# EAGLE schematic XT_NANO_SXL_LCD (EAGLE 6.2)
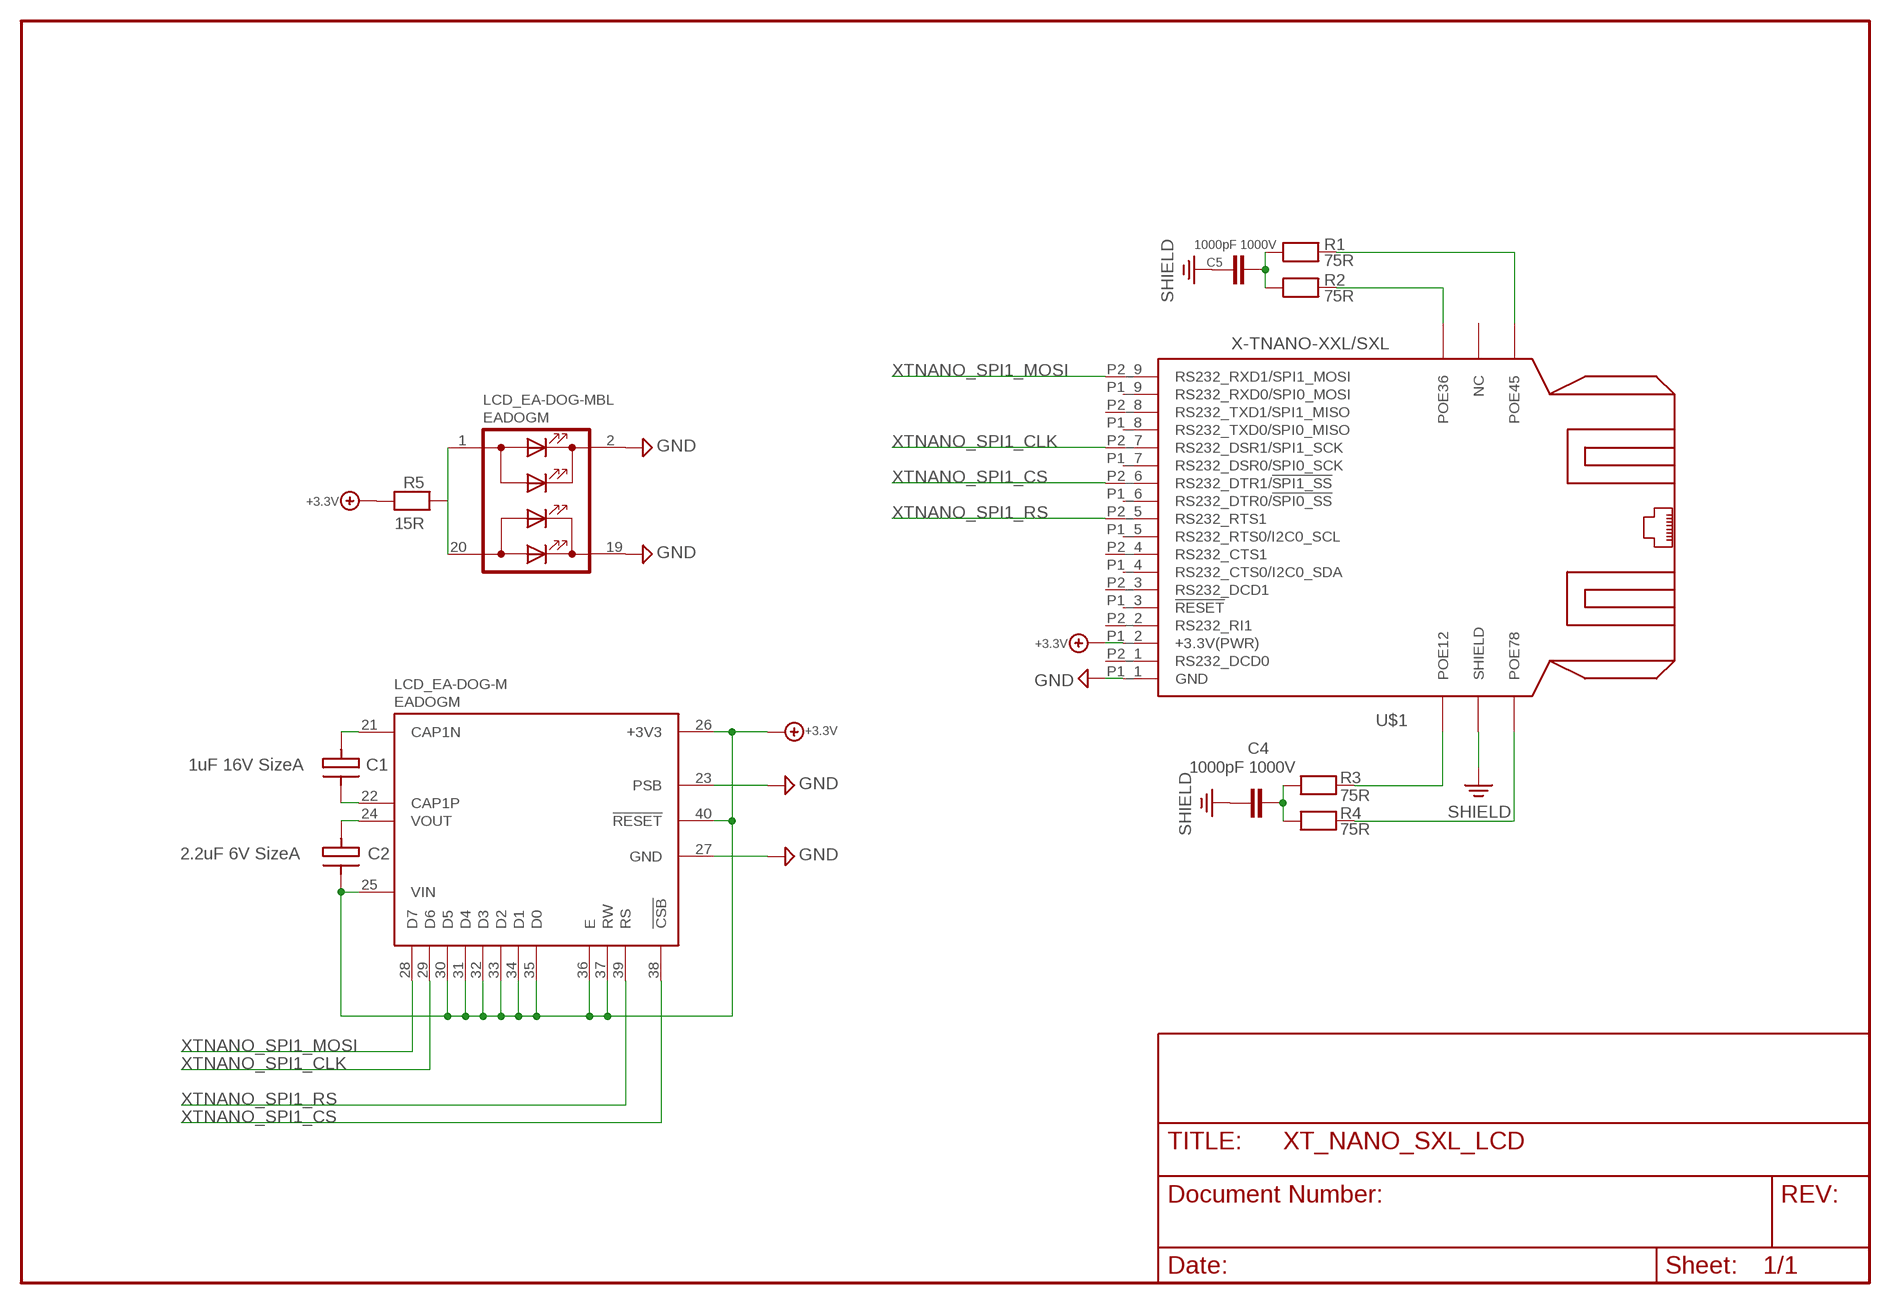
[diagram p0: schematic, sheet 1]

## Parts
C1  1uF 16V SizeA  C3216  [ORCAD_X_CT3216]
C2  2.2uF 6V SizeA  C3216  [ORCAD_X_CT3216]
C4  1000pF 1000V  CHIP-C-1210  [SMD-1210]
C5  1000pF 1000V  CHIP-C-1210  [SMD-1210]
LCD_EA-DOG-M  EADOGM  [EADOGM]
R1  75R  CHIP-R-0603  [SMD-0603]
R2  75R  CHIP-R-0603  [SMD-0603]
R3  75R  CHIP-R-0603  [SMD-0603]
R4  75R  CHIP-R-0603  [SMD-0603]
R5  15R  CHIP-R-0603  [SMD-0603]
U$1  X-TNANO-XXL/SXL  [XT-NANO-XXL/SXL]

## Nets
+3.3V: C2.2(C-) LCD_EA-DOG-M.25(VIN) LCD_EA-DOG-M.26(+3V3) LCD_EA-DOG-M.30(D5) LCD_EA-DOG-M.31(D4) LCD_EA-DOG-M.32(D3) LCD_EA-DOG-M.33(D2) LCD_EA-DOG-M.34(D1) LCD_EA-DOG-M.35(D0) LCD_EA-DOG-M.36(E) LCD_EA-DOG-M.37(RW) LCD_EA-DOG-M.40(!RESET) R5.1 U$1.P1_2(+3.3V(PWR))
GND: LCD_EA-DOG-M.2(C1) LCD_EA-DOG-M.19(C2) LCD_EA-DOG-M.23(PSB) LCD_EA-DOG-M.27(GND) U$1.P1_1(GND)
N$1: C5.1 R1.1 R2.1
N$2: C4.2 R3.1 R4.1
N$4: R2.2 U$1.POE36
N$5: LCD_EA-DOG-M.1(A1) LCD_EA-DOG-M.20(A2) R5.2
N$6: R1.2 U$1.POE45
N$7: C2.1(C+) LCD_EA-DOG-M.24(VOUT)
N$9: C1.2(C-) LCD_EA-DOG-M.22(CAP1P)
N$11: C1.1(C+) LCD_EA-DOG-M.21(CAP1N)
N$20: R3.2 U$1.POE12
N$21: R4.2 U$1.POE78
SHIELD: C4.1 C5.2 U$1.SHIELD
XTNANO_SPI1_CLK: LCD_EA-DOG-M.29(D6) U$1.P2_7(RS232_DSR1/SPI1_SCK)
XTNANO_SPI1_CS: LCD_EA-DOG-M.38(!CSB) U$1.P2_6(RS232_DTR1/!SPI1_SS!)
XTNANO_SPI1_MOSI: LCD_EA-DOG-M.28(D7) U$1.P2_9(RS232_RXD1/SPI1_MOSI)
XTNANO_SPI1_RS: LCD_EA-DOG-M.39(RS) U$1.P2_5(RS232_RTS1)
Unconnected: U$1.FLASH(NC) U$1.P1_3(!RESET) U$1.P1_4(RS232_CTS0/I2C0_SDA) U$1.P1_5(RS232_RTS0/I2C0_SCL) U$1.P1_6(RS232_DTR0/!SPI0_SS!) U$1.P1_7(RS232_DSR0/SPI0_SCK) U$1.P1_8(RS232_TXD0/SPI0_MISO) U$1.P1_9(RS232_RXD0/SPI0_MOSI) U$1.P2_1(RS232_DCD0) U$1.P2_2(RS232_RI1) U$1.P2_3(RS232_DCD1) U$1.P2_4(RS232_CTS1) U$1.P2_8(RS232_TXD1/SPI1_MISO)

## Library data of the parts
C1 C2 = XTMACRO:C3216
C4 C5 = XTMACRO:CHIP-C-?: Chip capacitance
LCD_EA-DOG-M = XTMACRO:EADOGM: THT EA LCD Display With LED Backlight
R1-R4 = XTMACRO:CHIP-R-?: Chip resistors
R5 = mea-lib:CHIP-R-?: Chip resistors
U$1 = ak-devices:X-TNANO-XXL/SXL: AK-NORD XT-NANO-XXL/SXL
